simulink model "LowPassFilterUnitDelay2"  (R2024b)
settings: Solver=FixedStepAuto  StartTime=0.0  StopTime=0.3  FixedStep=1e-3  RelTol=1e-3

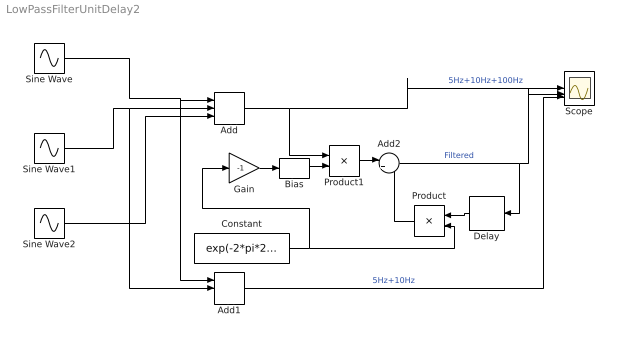
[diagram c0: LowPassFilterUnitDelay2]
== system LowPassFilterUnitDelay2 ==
  Add : Sum  Inputs=+++
  Add1 : Sum  Inputs=+++
  Add2 : Sum  Inputs=|++
  Bias : Bias  Bias=1
  Constant : Constant  Value=exp(-2*pi*20*1e-3)
  Delay : Delay  DelayLength=1
  Gain : Gain  Gain=-1
  Product : Product
  Product1 : Product
  Scope : Scope  NumInputPorts=3
  Sine Wave : Sin  Frequency=2 * pi * 5  SampleTime=0
  Sine Wave1 : Sin  Frequency=2 * pi * 10  Phase=pi/4  SampleTime=0
  Sine Wave2 : Sin  Frequency=2 * pi * 100  Phase=pi/2  SampleTime=0
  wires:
  Sine Wave/1 -> Add1/1, Add/1
  Sine Wave1/1 -> Add1/2, Add/2
  Sine Wave2/1 -> Add/3
  Add/1 -> Product1/1, Scope/1  "5Hz+10Hz+100Hz"
  Add1/1 -> Scope/3  "5Hz+10Hz"
  Product1/1 -> Add2/1
  Add2/1 -> Delay/1, Scope/2  "Filtered"
  Delay/1 -> Product/1
  Product/1 -> Add2/2
  Constant/1 -> Gain/1, Product/2
  Bias/1 -> Product1/2
  Gain/1 -> Bias/1
